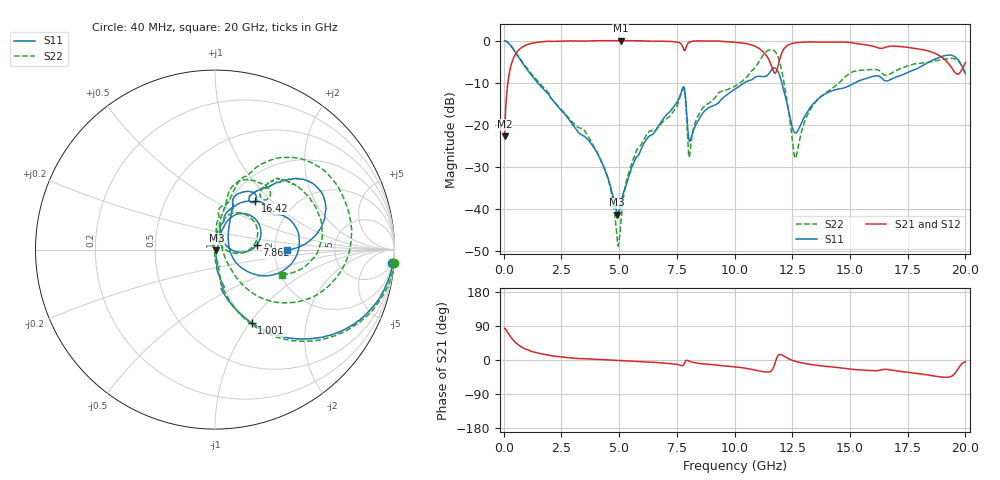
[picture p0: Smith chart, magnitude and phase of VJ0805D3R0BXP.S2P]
! VJ0805D3R0BXP
! DATE 10/29/2021  11:43
! CAPACITORS MOUNTED IN SERIES ON 25 MIL THICK MICROSTRIP SUBSTRATE
# GHz  S  MA  R  50.00
!  FREQ  S11M  S11A  S21M  S21A  S12M  S12A  S22M  S22A
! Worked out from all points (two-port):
!   1601 points, 40 MHz to 20 GHz, reference 50 ohm
!   highest |S21| = -0.02 dB at 5.067 GHz (marker M1); lowest = -22.7 dB at 40 MHz (marker M2)
!   |S21| within 3 dB of the highest: 535.8 MHz to 11.3 GHz (10.76 GHz wide, 182 % of centre); 12.04 GHz to 18.67 GHz (6.629 GHz wide, 43.2 % of centre)
!   lowest |S11| = -41.3 dB at 4.918 GHz (marker M3), VSWR 1.02, Z = 50.8 - j0.333 ohm
!   |S11| at or under -10 dB: 1.468 GHz to 10.44 GHz (8.971 GHz wide, 151 % of centre); 12.05 GHz to 15.22 GHz (3.176 GHz wide, 23.3 % of centre)
!   |S22| runs from -48.8 to 0.0 dB; largest |S21 - S12| = 0.0063
!   S11 on the Smith chart (normalised r, x): 40 MHz: 4, -27; 1.001 GHz: 0.99, -1.02; 7.862 GHz: 1.60, +0.08; 16.42 GHz: 1.30, +0.80; 20 GHz: 2.35, -0.02
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0.04  0.9901 -4.2  0.07331 83.7  0.0741 84.6  1.001 -4.3
0.3394  0.8438 -32.0  0.5313 57.9  0.5311 57.9  0.854 -32.3
1.000575  0.4577 -63.4  0.8906 27.4  0.8896 27.4  0.4736 -63.3
3.370825  0.07606 -78.6  0.9818 3.5  0.982 3.5  0.09086 -77.2
4.443675  0.02656 -76.5  0.9963 0.4  0.9952 0.5  0.02614 -93.4
4.917725  0.008628 -22.3  0.9968 -1.0  0.9975 -1.1  0.004389 -138.7
5.067425  0.01123 20.8  0.9981 -1.5  0.9978 -1.6  0.006471 133.4
5.6787  0.03784 56.8  0.9927 -3.5  0.993 -3.6  0.04377 96.2
6.70165  0.09698 69.2  0.9849 -6.8  0.9848 -6.9  0.09379 82.4
7.861825  0.2338 6.1  0.7745 -4.1  0.7747 -4.2  0.2165 6.1
8.0739  0.06435 40.0  0.9656 -4.1  0.9653 -4.2  0.04824 63.2
8.610325  0.1363 76.6  0.9877 -10.1  0.9877 -10.2  0.1562 85.4
10.02  0.2647 65.6  0.9512 -18.0  0.9505 -18.2  0.2874 74.0
11.23007  0.3736 33.6  0.7379 -30.7  0.7372 -30.8  0.6647 50.7
11.6667  0.466 15.8  0.4443 -22.3  0.4441 -22.4  0.7698 8.3
12.00352  0.3487 -24.0  0.6625 14.6  0.6625 14.3  0.4926 -37.0
12.62727  0.08038 8.9  0.9374 -3.4  0.9375 -3.5  0.04037 9.9
13.35083  0.1703 61.0  0.9597 -12.3  0.9598 -12.5  0.1631 80.1
16.41968  0.3492 50.3  0.8107 -25.1  0.8097 -25.4  0.4039 43.9
16.68165  0.3364 55.8  0.8519 -25.4  0.8522 -25.8  0.3937 50.7
18.7525  0.613 40.1  0.6909 -43.3  0.6897 -43.3  0.5774 37.8
20  0.4025 -0.5  0.5465 -5.0  0.5457 -5.2  0.3979 -20.5
